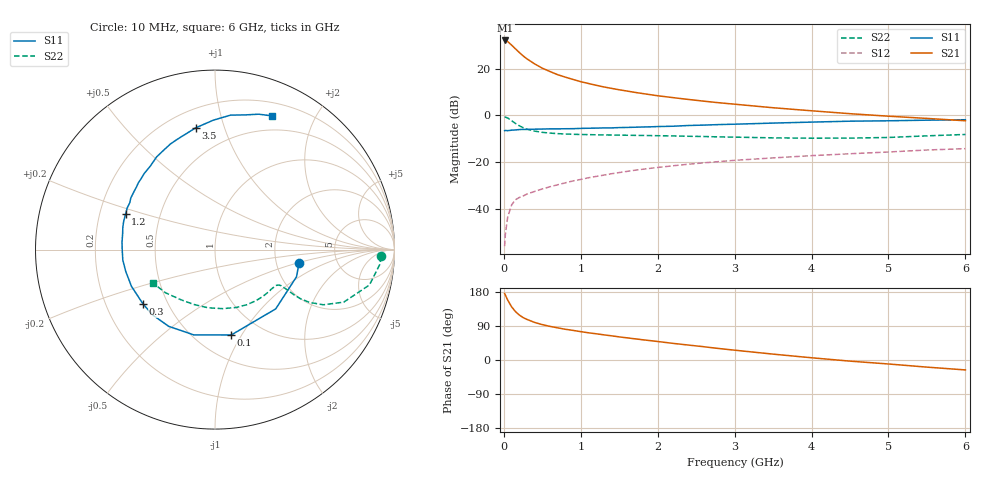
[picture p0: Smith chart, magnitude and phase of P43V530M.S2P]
! SIEMENS Small Signal Semiconductors
! BFP182
! Si NPN RF Bipolar Junction Transistor in SOT143
! VCE = 3.5 V  IC = 30 mA
! Common Emitter S-Parameters:  March  1996
# GHz  S  MA  R  50
!  f  S11  S21  S12  S22
! GHz  MAG  ANG  MAG  ANG  MAG  ANG  MAG  ANG
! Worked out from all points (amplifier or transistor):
!   36 points, 10 MHz to 6 GHz, reference 50 ohm
!   highest |S21| = 32.1 dB at 20 MHz (marker M1)
!   |S21| within 3 dB of that: start of sweep to 132.6 MHz
!   unconditionally stable (mu >= 1): 487.8 MHz to 5.61 GHz
!   at 250 MHz: K = 0.68, MSG = 30.0 dB, |S12| = -34.5 dB
!   at 1.4 GHz: K = 1.30, MAG = 15.0 dB, |S12| = -24.9 dB
!   at 6 GHz: K = 0.97, MSG = 6.0 dB, |S12| = -14.2 dB
!   S11 on the Smith chart (normalised r, x): 10 MHz: 2.69, -0.52; 100 MHz: 0.73, -0.90; 300 MHz: 0.36, -0.29; 1.2 GHz: 0.31, +0.18; 3.5 GHz: 0.31, +0.80; 6 GHz: 0.34, +1.46
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0.01  0.4739 -9.1  40.15 175.3  0.0016 81.6  0.9255 -2.3
0.02  0.4788 -18.4  40.2 171.2  0.0029 83.0  0.9222 -5.1
0.05  0.4728 -44.3  38.04 158.2  0.0067 75.9  0.8828 -12.9
0.1  0.4842 -79.2  32.08 140.6  0.0121 61.3  0.7747 -22.2
0.15  0.4897 -103.9  26.7 128.0  0.0157 54.9  0.6773 -27.0
0.2  0.4993 -121.1  22.31 118.8  0.0176 52.1  0.6026 -29.2
0.25  0.5031 -133.5  18.84 112.0  0.0189 51.3  0.5488 -29.9
0.3  0.5026 -143.0  16.26 107.1  0.0208 51.6  0.5099 -29.8
0.4  0.5085 -156.4  12.69 99.2  0.0237 53.1  0.4626 -29.2
0.5  0.5119 -166.3  10.26 93.3  0.0268 53.1  0.4355 -28.8
0.6  0.5169 -173.5  8.698 88.7  0.0299 54.9  0.4191 -28.6
0.7  0.5168 -179.5  7.445 84.8  0.0329 56.0  0.4086 -29.0
0.8  0.5198 175.4  6.597 81.1  0.0362 57.3  0.4015 -29.5
1.1  0.5329 162.5  4.828 71.8  0.0465 58.0  0.3888 -32.6
1.2  0.5361 158.1  4.42 69.2  0.0496 57.6  0.3858 -33.9
1.7  0.5597 141.4  3.123 56.0  0.0673 56.0  0.3753 -41.8
2.2  0.5884 127.8  2.406 43.9  0.0839 52.6  0.3648 -51.4
2.8  0.6387 112.9  1.867 30.2  0.1032 47.4  0.3477 -64.7
3.5  0.6869 99.0  1.462 15.5  0.1236 41.1  0.3316 -82.7
4.5  0.7542 83.4  1.091 -3.0  0.1517 32.2  0.3277 -111.3
5.5  0.7928 72.1  0.865 -18.8  0.1824 23.7  0.3663 -139.0
6  0.8102 66.8  0.77 -26.2  0.1949 18.5  0.3924 -151.8
